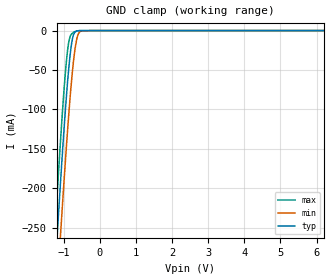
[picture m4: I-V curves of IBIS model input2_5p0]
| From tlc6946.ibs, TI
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|   input2_5p0 Model
[Model]   input2_5p0
Model_type   Input
Vinl = 1.5
Vinh = 3.5
|   typ   min   max
C_comp   1.3666pF   1.3479pF   1.3856pF
|  Where Nom  PVT is Nominal Process, 5.0V,   27C
|   Fast PVT is Strong Process,  5.5V,   -40C
|   Slow PVT is Weak Process,   4.5V,   105C
[Model spec]
|subparameter
Vinl   1.5   1.35   1.65
Vinh   3.5   3.15   3.85
[Voltage Range]   5   4.5   5.5
|Junction Temperature
[Temperature Range]   27   105   -40
[Power Clamp Reference]   5   4.5   5.5
[GND Clamp Reference]   0   0   0
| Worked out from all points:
|   GND clamp passes 1 mA (typ) near -0.66 V on its own axis
[GND Clamp]
|   Voltage   I(typ)   I(min)   I(max)
-3V       -1.709A    -1.711A    -1.711A
-1.251V   -312.6mA   -378.3mA   -260.9mA
-1.24V    -304.2mA   -370mA     -252.4mA
-1.185V   -262.6mA   -329mA     -210.1mA
-1.086V   -189.9mA   -256.8mA   -137.3mA
-987mV    -121.7mA   -187.5mA   -71.84mA
-910mV    -74.04mA   -136.7mA   -31.57mA
-800mV    -21.98mA   -71.89mA   -5.356mA
-690mV    -1.834mA   -23.96mA   -1.292mA
-580mV    -112uA     -2.779mA   -132.3uA
-239mV    0A         -108.1nA   0A
8V        0A         0A         0A
[POWER Clamp]
|   Voltage   I(typ)   I(min)   I(max)
-3V       0A         0A         0A
8V        0A         0A         0A
